(* Logix 5000 Rung export; software revision 16.04 *)

MODULES
   Local : vendor None type None code None
   SIE : vendor None type None code None
END_MODULES

TYPE SIEIPADDRESS :   // Data structure to get and set the IP address of the module.
STRUCT
   IPGetTrigger : BOOL;   // Gets IP Address
   IPReceived : INT[4];   // IP address received.
   IPSetTrigger : BOOL;   // Sets IP Address
   IPRequested : INT[4];   // IP address set.
END_STRUCT
END_TYPE

TYPE SIEMODULEDEF :   // This defines the whole module which includes all tags used in the program
STRUCT
   DATA : SIEDATA;   // Data read from module
   CONTROL : SIECONTROL;   // Client ,Server Status and blocks status
   STATUS : SIESTATUS;   // SIE Module control
   UTIL : SIEUTIL;   // Block statistics
END_STRUCT
END_TYPE

TYPE SIEBLOCKSTATS :   // This object is used to store the block transfer statistics for the MVI56E-SIE module.
STRUCT
   Read : INT;   // Total number of read block transfers
   Write : INT;   // Total number of write block transfers
   Parse : INT;   // Total number of blocks parsed
   Reserved : INT;   // Used internally for future use
   Cmd : INT;   // Total number of command blocks received
   Err : INT;   // Total number of block transfer errors
END_STRUCT
END_TYPE

TYPE SIEDATA :   // Contains Read Data (data read from the module to the processor) and Write Data (data written from the processor to the module)
STRUCT
   ReadData : INT[600];   // Data read from module. Set array equal to the size set in the Configuration file.
   WriteData : INT[600];   // Data to write to module. Set array equal to the size set in the Configuration file.
END_STRUCT
END_TYPE

TYPE SIECLIENTSTATS :   // This object is used to store the port statistics for an MVI56E-SIE port.
STRUCT
   CmdReq : INT;   // Total number of command list requests sent
   CmdResp : INT;   // Total number of command list responses received
   CmdErr : INT;   // Total number of command list errors
   Requests : INT;   // Total number of requests for port
   Responses : INT;   // Total number of responses for port
   ErrSent : INT;   // Total number of errors sent
   ErrRec : INT;   // Total number of errors received
   CfgErrWord : INT;   // Configuration Error Word
   CurErr : INT;   // Current Error code
   LastErr : INT;   // Last recorded error code
END_STRUCT
END_TYPE

TYPE SIESTATUS :   // This status data is returned on each read block and can be used to detect proper module operation.
STRUCT
   PassCnt : INT;   // Program cycle counter
   ProductVersion : INT;   // This is used to pass the product version to the processor
   ProductCode : INT[2];   // This is used to pass the product Code to the processor
   BlockStats : SIEBLOCKSTATS;   // Block transfer statistics
   CmdBits : INT[20];   // Commands bits array to be used for 20 clients
   ClientStatsTrigger : BOOL;   // Get Client Status
   ClientID : INT;   // Client ID to get Status From
   ClientStatus : SIECLIENTSTATS[20];   // Client status data
   CmdErrorList : INT[16];   // Command Error List
END_STRUCT
END_TYPE

TYPE SIECONTROL :   // Values used by program for data transfer operation between the module and the processor.
STRUCT
   BootTimer : TIMER;   // Timer used to clear both cold and warm boot requests
   ColdBoot : BOOL;   // Hardware reset of the Module
   WarmBoot : BOOL;   // Configuration data reset in the Module.
   ResetStatus : BOOL;   // Resets module status
   CmdID : INT;   // Command ID from 1 to 16
   CmdControl : SIECMDCONTROL;   // Holds Command Control statistics
   CmdControlPending : BOOL;   // Halts rung until Module is ready.
   CmdControlTrigger : BOOL;   // Command Control Trigger
   IPAddress : SIEIPADDRESS;   // Getting and Setting IP address to and from Module
END_STRUCT
END_TYPE

TYPE SIEINITOUTDATA :   // Used to bring the Module into a known state after a restart operation.
STRUCT
   InitOutBlkIDLim : INT;   // Block Index Limit for ReadData size of the array
END_STRUCT
END_TYPE

TYPE SIECMDCONTROL :   // MVI56E-SIE Command Control
STRUCT
   ClientID : INT;   // Block5000 Client Identification by Index number 0 to 19
   CMDqty : INT;   // Block5000 command quantity
   CmdIndex : INT[16];   // Contains index in the command list for the 1st command to be entered into Command queue
   WriteCmdBits : INT[20];   // Command Bit control ClientID(0 to 19)
END_STRUCT
END_TYPE

TYPE SIEUTIL :   // Values used by program for data transfer operation between the module and the processor.
STRUCT
   LastRead : INT;   // Index of last read block
   LastWrite : INT;   // Index of last write block
   BlockIndex : INT;   // Computed block offset for data table
   StatusIndex : INT;   // Computed block offset for status data
   ReadDataSizeGet : INT;   // Gets ReadData Array Length.
   WriteDataSizeGet : INT;   // Gets WriteData Array Length.
   ReadDataBlkCount : INT;   // Holds the value of the Block Counts of the Read Data Array.
   WriteDataBlkCount : INT;   // Holds the value of the Block Counts of the Write Data Array.
   RBTSremainder : INT;   // Holds remainder calculation value from the read array.
   WBTSremainder : INT;   // Holds remainder calculation value from the write array.
   IPsetPending : BOOL;   // Allows Setting module IP address
   IPgetPending : BOOL;   // Allows Getting module IP address
   InitOutputData : SIEINITOUTDATA;
   CheckInitialization : BOOL;   // Check Initialization trigger
   StatusSeqIndex : INT;   // Computed block offset for status data
END_STRUCT
END_TYPE

ADD_ON_INSTRUCTION AOI56ESIE   (* revision 1.2, vendor Prosoft Technology, Inc, ExecutePrescan *)
// MVI56E-SIE AddOn_Rung
// Revision note:
// v1_2 Fix to Memory Overflow bug in several Instructions
VAR_IN_OUT
   Connection_Input : INT[250]; {required}   // Input parameters.
   Connection_Output : INT[248]; {required}   // Output parameters.
   SIE : SIEMODULEDEF; {required}
END_VAR
VAR
   MJFAULTS : DINT[12];
END_VAR

ROUTINE Logic   (* ladder *)
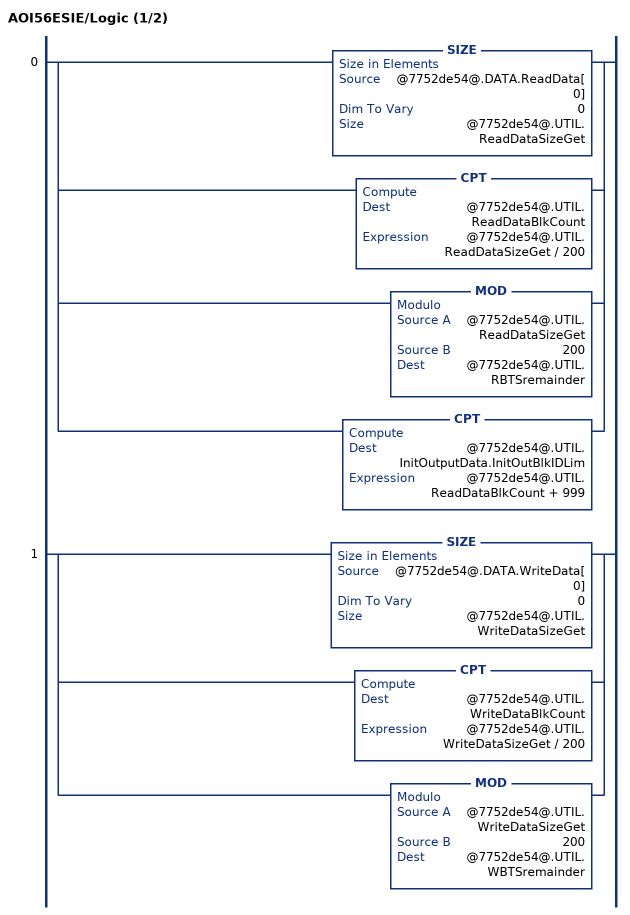
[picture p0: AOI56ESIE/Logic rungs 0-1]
   0: [SIZE(@7752de54@.DATA.ReadData[0],0,@7752de54@.UTIL.ReadDataSizeGet) ,CPT(@7752de54@.UTIL.ReadDataBlkCount,@7752de54@.UTIL.ReadDataSizeGet / 200) ,MOD(@7752de54@.UTIL.ReadDataSizeGet,200,@7752de54@.UTIL.RBTSremainder) ,CPT(@7752de54@.UTIL.InitOutputData.InitOutBlkIDLim,@7752de54@.UTIL.ReadDataBlkCount + 999) ];
   1: [SIZE(@7752de54@.DATA.WriteData[0],0,@7752de54@.UTIL.WriteDataSizeGet) ,CPT(@7752de54@.UTIL.WriteDataBlkCount,@7752de54@.UTIL.WriteDataSizeGet / 200) ,MOD(@7752de54@.UTIL.WriteDataSizeGet,200,@7752de54@.UTIL.WBTSremainder) ];
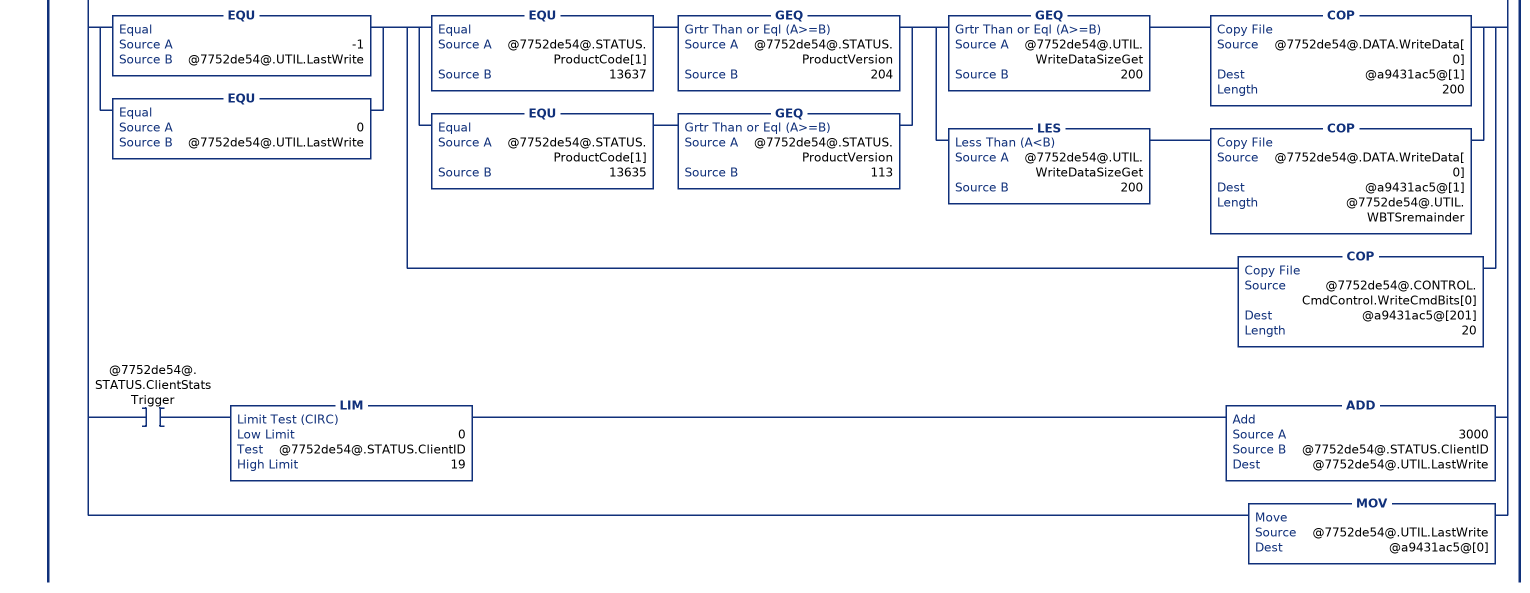
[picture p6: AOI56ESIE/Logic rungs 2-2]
   2: NEQ(@0dfc57aa@[249],@7752de54@.UTIL.LastRead)[MOV(@0dfc57aa@[249],@7752de54@.UTIL.LastRead) ,GEQ(@7752de54@.UTIL.LastRead,1) [LEQ(@7752de54@.UTIL.LastRead,@7752de54@.UTIL.ReadDataBlkCount) [CPT(@7752de54@.UTIL.BlockIndex,(@7752de54@.UTIL.LastRead-1)*200) ,COP(@0dfc57aa@[2],@7752de54@.DATA.ReadData[@7752de54@.UTIL.BlockIndex],200) ,COP(@0dfc57aa@[202],@7752de54@.STATUS.PassCnt,1) ,COP(@0dfc57aa@[203],@7752de54@.STATUS.BlockStats.Read,6) ,COP(@0dfc57aa@[209],@7752de54@.STATUS.CmdBits[0],20) ,COP(@0dfc57aa@[229],@7752de54@.STATUS.ProductCode[0],2) ,COP(@0dfc57aa@[231],@7752de54@.STATUS.ProductVersion,1) ] ,CMP(@7752de54@.UTIL.LastRead - @7752de54@.UTIL.ReadDataBlkCount = 1) GRT(@7752de54@.UTIL.RBTSremainder,0) [CPT(@7752de54@.UTIL.BlockIndex,(@7752de54@.UTIL.LastRead - 1) * 200) ,COP(@0dfc57aa@[2],@7752de54@.DATA.ReadData[@7752de54@.UTIL.BlockIndex],@7752de54@.UTIL.RBTSremainder) ,COP(@0dfc57aa@[202],@7752de54@.STATUS.PassCnt,1) ,COP(@0dfc57aa@[203],@7752de54@.STATUS.BlockStats.Read,6) ,COP(@0dfc57aa@[209],@7752de54@.STATUS.CmdBits[0],20) ,COP(@0dfc57aa@[229],@7752de54@.STATUS.ProductCode[0],2) ,COP(@0dfc57aa@[231],@7752de54@.STATUS.ProductVersion,1) ] ] ,LIM(3000,@7752de54@.UTIL.LastRead,3029) [CPT(@7752de54@.UTIL.StatusIndex,@7752de54@.UTIL.LastRead-3000) ,COP(@0dfc57aa@[3],@7752de54@.STATUS.ClientStatus[@7752de54@.UTIL.StatusIndex].CmdReq,10) ,COP(@0dfc57aa@[13],@7752de54@.STATUS.CmdErrorList[0],16) ,OTU(@7752de54@.STATUS.ClientStatsTrigger) ] ,EQU(@7752de54@.UTIL.LastRead,9990) [COP(@0dfc57aa@[2],@7752de54@.CONTROL.IPAddress.IPRequested[0],4) ,OTU(@7752de54@.UTIL.IPsetPending) ] ,EQU(@7752de54@.UTIL.LastRead,9991) [COP(@0dfc57aa@[2],@7752de54@.CONTROL.IPAddress.IPReceived[0],4) ,OTU(@7752de54@.UTIL.IPgetPending) ] ,XIC(@7752de54@.CONTROL.CmdControlTrigger) LIM(5001,@7752de54@.UTIL.LastRead,5016) LIM(1,@0dfc57aa@[2],16) OTU(@7752de54@.CONTROL.CmdControlTrigger) ,MOV(@0dfc57aa@[1],@7752de54@.UTIL.LastWrite) ,XIC(@7752de54@.CONTROL.WarmBoot) [MOV(9998,@7752de54@.UTIL.LastWrite) ,OTU(@7752de54@.CONTROL.WarmBoot) ] ,XIC(@7752de54@.CONTROL.ColdBoot) [MOV(9999,@7752de54@.UTIL.LastWrite) ,OTU(@7752de54@.CONTROL.ColdBoot) ] ,XIC(@7752de54@.CONTROL.ResetStatus) [MOV(9997,@7752de54@.UTIL.LastWrite) ,OTU(@7752de54@.CONTROL.ResetStatus) ] ,XIC(@7752de54@.CONTROL.IPAddress.IPSetTrigger) XIO(@7752de54@.UTIL.IPsetPending) [COP(@7752de54@.CONTROL.IPAddress.IPRequested[0],@a9431ac5@[1],4) ,MOV(9990,@7752de54@.UTIL.LastWrite) ,OTU(@7752de54@.CONTROL.IPAddress.IPSetTrigger) ,OTL(@7752de54@.UTIL.IPsetPending) ] ,XIC(@7752de54@.CONTROL.IPAddress.IPGetTrigger) XIO(@7752de54@.UTIL.IPgetPending) [MOV(9991,@7752de54@.UTIL.LastWrite) ,OTU(@7752de54@.CONTROL.IPAddress.IPGetTrigger) ,OTL(@7752de54@.UTIL.IPgetPending) ] ,XIC(@7752de54@.CONTROL.CmdControlTrigger) LIM(1,@7752de54@.CONTROL.CmdID,16) [LIM(0,@7752de54@.CONTROL.CmdControl.ClientID,19) MOV(@7752de54@.CONTROL.CmdControl.ClientID,@a9431ac5@[1]) ,COP(@7752de54@.CONTROL.CmdControl.CmdIndex[0],@a9431ac5@[2],16) ,ADD(5000,@7752de54@.CONTROL.CmdID,@7752de54@.UTIL.LastWrite) ] ,GEQ(@7752de54@.UTIL.LastWrite,1) [LEQ(@7752de54@.UTIL.LastWrite,@7752de54@.UTIL.WriteDataBlkCount) [CPT(@7752de54@.UTIL.BlockIndex,(@7752de54@.UTIL.LastWrite-1)*200) ,COP(@7752de54@.DATA.WriteData[@7752de54@.UTIL.BlockIndex],@a9431ac5@[1],200) ,COP(@7752de54@.CONTROL.CmdControl.WriteCmdBits[0],@a9431ac5@[201],20) ] ,CMP(@7752de54@.UTIL.LastWrite - @7752de54@.UTIL.WriteDataBlkCount = 1) GRT(@7752de54@.UTIL.WBTSremainder,0) [CPT(@7752de54@.UTIL.BlockIndex,(@7752de54@.UTIL.LastWrite - 1) * 200) ,COP(@7752de54@.DATA.WriteData[@7752de54@.UTIL.BlockIndex],@a9431ac5@[1],@7752de54@.UTIL.WBTSremainder) ,COP(@7752de54@.CONTROL.CmdControl.WriteCmdBits[0],@a9431ac5@[201],20) ] ] ,LIM(1000,@7752de54@.UTIL.LastWrite,1024) LEQ(@7752de54@.UTIL.LastWrite,@7752de54@.UTIL.InitOutputData.InitOutBlkIDLim) [CPT(@7752de54@.UTIL.BlockIndex,(@7752de54@.UTIL.LastWrite-1000)*200) ,COP(@7752de54@.DATA.ReadData[@7752de54@.UTIL.BlockIndex],@a9431ac5@[1],200) ] ,[EQU(-1,@7752de54@.UTIL.LastWrite) ,EQU(0,@7752de54@.UTIL.LastWrite) ] [[EQU(@7752de54@.STATUS.ProductCode[1],13637) GEQ(@7752de54@.STATUS.ProductVersion,204) ,EQU(@7752de54@.STATUS.ProductCode[1],13635) GEQ(@7752de54@.STATUS.ProductVersion,113) ] [GEQ(@7752de54@.UTIL.WriteDataSizeGet,200) COP(@7752de54@.DATA.WriteData[0],@a9431ac5@[1],200) ,LES(@7752de54@.UTIL.WriteDataSizeGet,200) COP(@7752de54@.DATA.WriteData[0],@a9431ac5@[1],@7752de54@.UTIL.WBTSremainder) ] ,COP(@7752de54@.CONTROL.CmdControl.WriteCmdBits[0],@a9431ac5@[201],20) ] ,XIC(@7752de54@.STATUS.ClientStatsTrigger) LIM(0,@7752de54@.STATUS.ClientID,19) ADD(3000,@7752de54@.STATUS.ClientID,@7752de54@.UTIL.LastWrite) ,MOV(@7752de54@.UTIL.LastWrite,@a9431ac5@[0]) ];
END_ROUTINE

ROUTINE Prescan   (* ladder *)
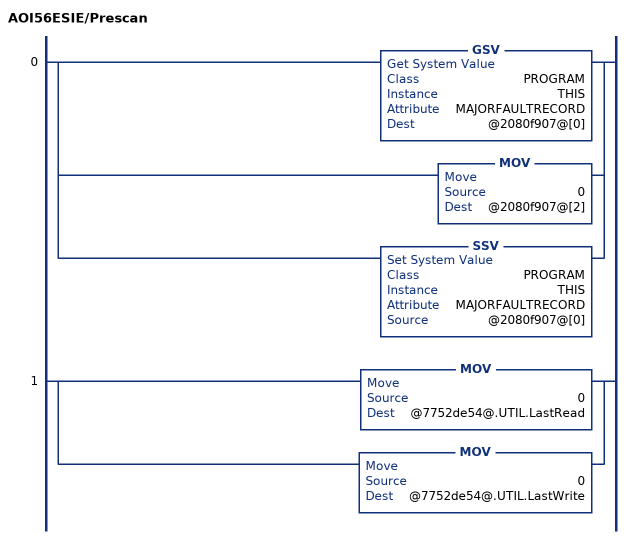
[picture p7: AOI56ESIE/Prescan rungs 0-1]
   0: [GSV(PROGRAM,THIS,MAJORFAULTRECORD,@2080f907@[0]) ,MOV(0,@2080f907@[2]) ,SSV(PROGRAM,THIS,MAJORFAULTRECORD,@2080f907@[0]) ];
   1: [MOV(0,@7752de54@.UTIL.LastRead) ,MOV(0,@7752de54@.UTIL.LastWrite) ];
END_ROUTINE
END_ADD_ON_INSTRUCTION

VAR_GLOBAL   (* controller tags *)
   AOI56SIE : AOI56ESIE;   // MVI56E-SIE AddOn_Rung
   SIE : SIEMODULEDEF;
   Local:1:I : AB:1756_MODULE_INT_500Bytes:I:0;
   Local:1:O : AB:1756_MODULE_INT_496Bytes:O:0;
END_VAR

PROGRAM MainProgram

ROUTINE MainRoutine   (* ladder *)
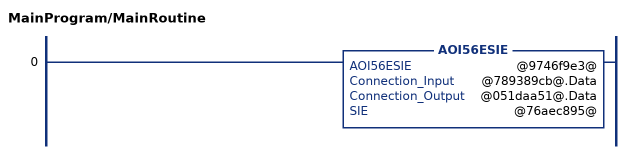
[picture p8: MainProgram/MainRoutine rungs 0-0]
   0: AOI56ESIE(@9746f9e3@,@789389cb@.Data,@051daa51@.Data,@76aec895@);
END_ROUTINE
END_PROGRAM
